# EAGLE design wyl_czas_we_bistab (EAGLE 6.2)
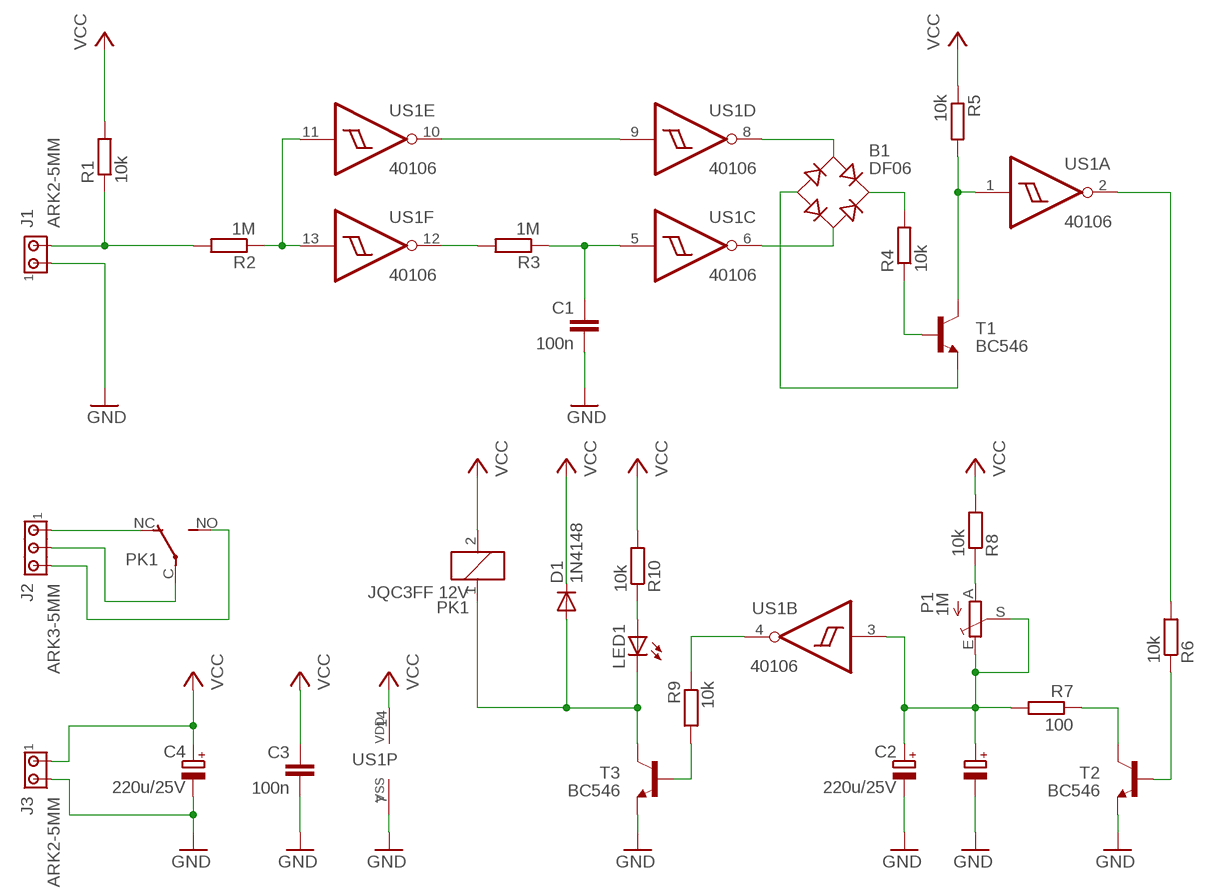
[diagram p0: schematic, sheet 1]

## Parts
B1  DF06  B-DIL  [B-DIL]
C1  100n  C-EU050-025X075  [C050-025X075]
C2  220u/25V  CPOL-EUE2.5-7  [E2,5-7]
C2'  CPOL-EUE5-10.5  [E5-10,5]
C3  100n  C-EU050-025X075  [C050-025X075]
C4  220u/25V  CPOL-EUE2.5-7  [E2,5-7]
D1  1N4148  1N4148DO35-7  [DO35-7]
J1  ARK2-5MM  [2PIN-5MM]
J2  ARK3-5MM  [3PIN-5MM]
J3  ARK2-5MM  [2PIN-5MM]
LED1  LED5MM  [LED5MM]
P1  1M  TRIM_EU-CA6V  [CA6V]
PK1  JQC3FF 12V  PK_POJED-JQC-3FG  [PK_POJED_JQC-3FG]
R1  10k  R-EU_0207/7  [0207/7]
R2  1M  R-EU_0207/7  [0207/7]
R3  1M  R-EU_0207/7  [0207/7]
R4  10k  R-EU_0207/2V  [0207/2V]
R5  10k  R-EU_0207/7  [0207/7]
R6  10k  R-EU_0207/2V  [0207/2V]
R7  100  R-EU_0207/2V  [0207/2V]
R8  10k  R-EU_0207/10  [0207/10]
R9  10k  R-EU_0207/2V  [0207/2V]
R10  10k  R-EU_0207/7  [0207/7]
T1  BC546  BC546B  [TO92-EBC]
T2  BC546  BC546B  [TO92-EBC]
T3  BC546  BC546B  [TO92-EBC]
US1  40106  40106N  [DIL14]

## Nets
GND: C1.2 C2'.- C2.- C3.2 C4.- J1.P$1 J3.P$2 T2.E T3.E US1.7(P:VSS)
J2: J2.P$2 PK1.C(COM)
N$1: B1.AC1 US1.8(D:O)
N$2: B1.+ R4.2
N$3: B1.AC2 US1.6(C:O)
N$4: R9.1 US1.4(B:O)
N$5: R4.1 T1.B
N$6: J1.P$2 R1.1 R2.2
N$7: R9.2 T3.B
N$8: LED1.A R10.1
N$9: J2.P$1 PK1.NC
N$10: R2.1 US1.11(E:I) US1.13(F:I)
N$11: J2.P$3 PK1.NO
N$12: R3.2 US1.12(F:O)
N$13: C1.1 R3.1 US1.5(C:I)
N$14: B1.- T1.E
N$15: R5.2 T1.C US1.1(A:I)
N$16: US1.9(D:I) US1.10(E:O)
N$17: R6.2 US1.2(A:O)
N$18: R6.1 T2.B
N$19: R7.1 T2.C
N$20: C2'.+ C2.+ P1.E P1.S R7.2 US1.3(B:I)
N$21: P1.A R8.1
N$22: D1.A LED1.K(C) PK1.1 T3.C
VCC: C3.1 C4.+ D1.C J3.P$1 PK1.2 R1.2 R5.1 R8.2 R10.2 US1.14(P:VDD)

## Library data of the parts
B1 = rectifier:B-DIL: RECTIFIER
C1 C3 = rcl:C-EU: CAPACITOR, European symbol
C2 C2' C4 = rcl:CPOL-EU: POLARIZED CAPACITOR, European symbol
D1 = diode:1N4148: DIODE
J1 J3 = zlacza_futrzak:ARK2: ARK 2
J2 = zlacza_futrzak:ARK3: ARK 3 Raster 5mm i 3,5mm
LED1 = led:LED: LED
P1 = pot:TRIM_EU-: POTENTIOMETER
PK1 = inne_futrzak:PK_POJED
R1-R10 = rcl:R-EU_: RESISTOR, European symbol
T1-T3 = transistor-npn:BC546*: NPN Transistor
US1 = 40xx:40106: Hex SCHMITT TRIGGER

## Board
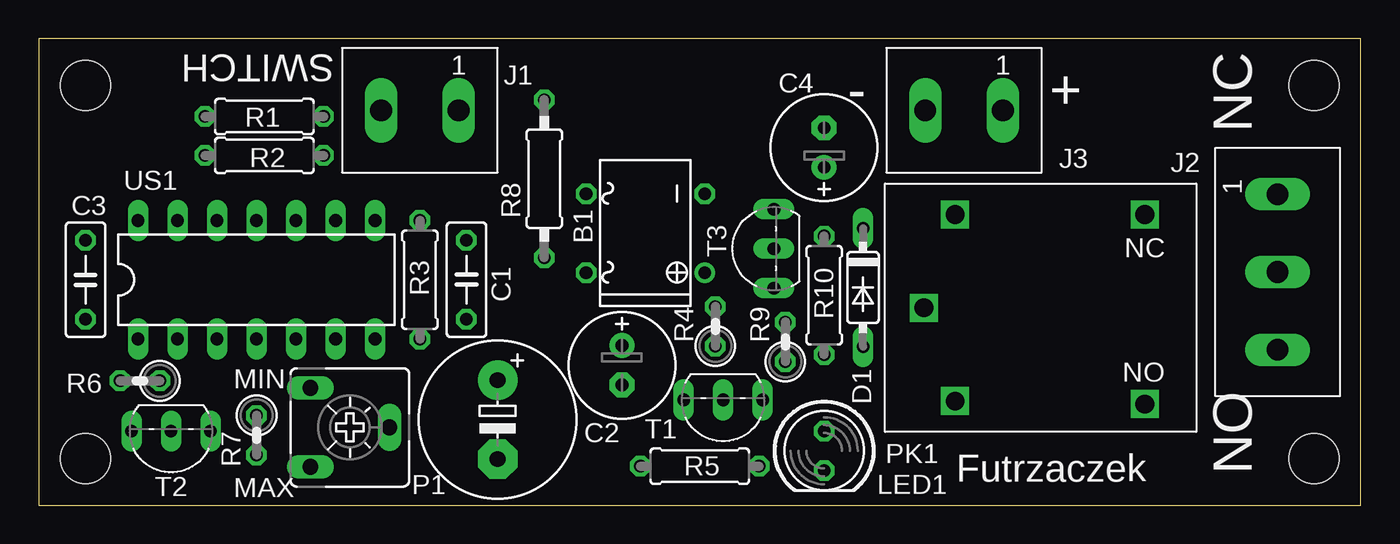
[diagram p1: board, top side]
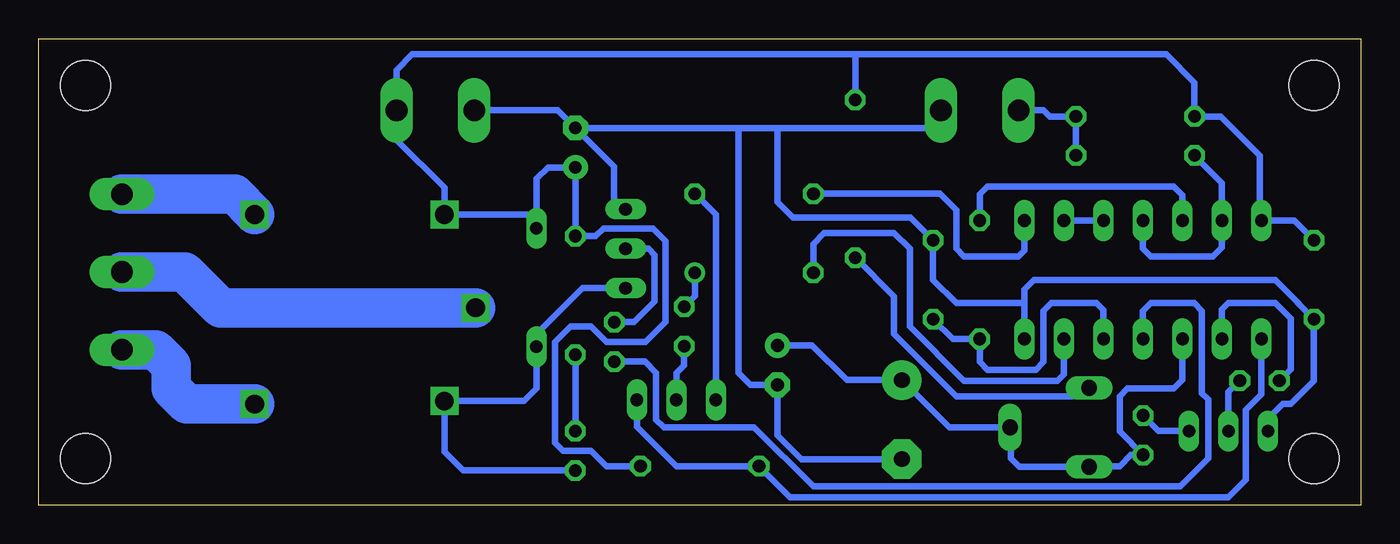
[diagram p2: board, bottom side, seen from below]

Size 85 x 30 mm. Coordinates in mm from the lower left corner, seen from the top.
Outline: 0,0 85,0 85,30 0,30 0,0
Copper layers (1*16): Top 0.035mm / dielectric 1.5mm / Bottom 0.035mm
Design rules: minimum track width 10mil, minimum drill 23mil, track to track 8mil, track to pad 8mil, pad to pad 8mil, via to via 8mil, smd to smd 8mil, copper to edge 10mil, drill to drill 8mil, minimum pad ring 10mil, minimum via ring 8mil, stop-mask expansion 4mil, vias tented up to drill 0mil, thermal gap 10mil
Holes 3.2 mm at 3,3 3,27 82,3 82,27

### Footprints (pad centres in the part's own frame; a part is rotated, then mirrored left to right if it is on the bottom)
B-DIL = drill 0.813: + -2.54,-3.81 | drill 0.813 octagon: - 2.54,-3.81; AC1 2.54,3.81; AC2 -2.54,3.81
C050-025X075 = drill 0.813 octagon: 1 -2.54,0; 2 2.54,0
E2,5-7 = drill 0.813 pad 1.6: + -1.27,0 | drill 0.813 pad 1.6 octagon: - 1.27,0
E5-10,5 = drill 1.016 pad 2.54: + -2.54,0 | drill 1.016 pad 2.54 octagon: - 2.54,0
DO35-7 = drill 0.813 long: A 3.81,0; C -3.81,0
2PIN-5MM = drill 1.4 long: P$1 -2.5,0; P$2 2.5,0
3PIN-5MM = drill 1.4 long: P$1 -5,0; P$2 0,0; P$3 5,0
LED5MM = drill 0.813 octagon: A -1.27,0; K 1.27,0
CA6V = drill 1.016 long: A -2.54,-2.54; E 2.54,-2.54; S 0,2.54
PK_POJED_JQC-3FG = drill 1.2 square: 1 5.5,6; 2 5.5,-6; C 7.5,0; NC -6.7,-6; NO -6.7,6.2
0207/7 = drill 0.813 octagon: 1 -3.81,0; 2 3.81,0
0207/2V = drill 0.813 octagon: 1 -1.27,0; 2 1.27,0
0207/10 = drill 0.813 octagon: 1 -5.08,0; 2 5.08,0
TO92-EBC = drill 0.813 long: B 0,-1.27; C -2.54,-1.27; E 2.54,-1.27
DIL14 = drill 0.813 long: 1 -7.62,-3.81; 2 -5.08,-3.81; 3 -2.54,-3.81; 4 0,-3.81; 5 2.54,-3.81; 6 5.08,-3.81; 7 7.62,-3.81; 8 7.62,3.81; 9 5.08,3.81; 10 2.54,3.81; 11 0,3.81; 12 -2.54,3.81; 13 -5.08,3.81; 14 -7.62,3.81

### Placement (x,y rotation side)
B1  39,17.5 90 top
C1  27.5,14.5 90 top
C2  37.5,9 270 top
C2'  29.5,5.5 270 top
C3  3,14.5 270 top
C4  50.5,23 90 top
D1  53,14 270 top
J1  24.5,25.4 180 top
J2  79.66,15 270 top
J3  59.5,25.4 180 top
LED1  50.5,3.5 270 top
P1  20,5 270 top
PK1  64.42,12.7 180 top
R1  14.5,25 180 top
R2  14.5,22.5 0 top
R3  24.5,14.5 90 top
R4  43.5,11.5 90 top
R5  42.5,2.5 180 top
R6  6.5,8 180 top
R7  14,4.5 270 top
R8  32.5,21 90 top
R9  48,10.5 90 top
R10  50.5,13.5 90 top
T1  44,5.5 180 top
T2  8.5,3.5 180 top
T3  46,16.5 90 top
US1  14,14.5 0 top

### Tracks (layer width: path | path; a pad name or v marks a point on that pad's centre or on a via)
GND
  Bottom 0.406: J1.P$1 27,24.5 27.5,24.5 27.77,24.27 37.5,24.27 | T3.E 47.54,19.04 48,19.5 48,21.77 C4.- | US1.7 21.62,13 | 21.62,13 26,13 27.5,14.5 C1.2 28.96,18.5 36.5,18.5 37.5,19.5 37.5,22.64 37.5,24.27 | 21.62,13 21.62,13.88 21,14.5 5.5,14.5 4,13 4.04,13 C3.2 3,8 4.5,6.5 5,6.5 5.96,5.54 T2.E | C2'.- 35.96,2.96 37.5,4.5 C2.- 39.23,7.73 40,8.5 40,23.14 40,24.27 | C4.- 40,24.27 | 40,24.27 37.5,24.27 | J3.P$2 51.63,25.4 C4.-
J2
  Bottom 2.54: PK1.C 73.31,12.7 75.61,15 J2.P$2
N$1
  Bottom 0.406: US1.8 21.62,16.38 22,16 25.5,16 26,16.5 26,19 27.04,20.04 B1.AC1
N$2
  Bottom 0.406: B1.+ 42.81,13.46 R4.2
N$3
  Bottom 0.406: US1.6 19.08,8.42 19.5,8 25.5,8 29,11.5 29,16.5 30,17.5 34.5,17.5 35.19,16.81 B1.AC2
N$4
  Bottom 0.406: US1.4 14,12.5 13.5,13 10.7,13 10.2,12.5 10.2,7.2 9.8,6.8 9.8,3 11.6,1.2 35.2,1.2 39,5 44.8,5 45.3,5.5 45.3,8.5 46.03,9.23 R9.1
N$5
  Bottom 0.406: T1.B 44,8.5 43.5,9 R4.1
N$6
  Bottom 0.406: J1.P$2 20.4,25.4 20,25 R1.1 R2.2
N$7
  Bottom 0.406: T3.B 45.8,16.5 45.4,16.1 45.4,13.1 46.73,11.77 R9.2
N$8
  Bottom 0.406: LED1.A R10.1
N$9
  Bottom 2.54: J2.P$1 72.42,20 PK1.NC
N$10
  Bottom 0.406: R2.1 8.92,20.73 US1.13 8.92,16.58 9.5,16 13.5,16 14,16.5 US1.11
N$11
  Bottom 2.54: PK1.NO 75.5,6.5 76.5,7.5 76.5,9 77.5,10 J2.P$3
N$12
  Bottom 0.406: R3.2 24.5,20 24,20.5 12,20.5 11.46,19.96 US1.12
N$13
  Bottom 0.406: C1.1 26.23,10.69 R3.1 24.5,9.2 24,8.7 20.9,8.7 20.4,9.2 20.4,12.5 19.9,13 17,13 16.54,12.54 US1.5
N$14
  Bottom 0.406: T1.E 41.46,18.69 B1.-
N$15
  Bottom 0.406: T1.C 46.54,5.04 44,2.5 R5.2 36.69,0.5 8.5,0.5 7.38,1.62 7.38,6.12 6.38,7.12 US1.1
N$16
  Bottom 0.406: US1.10 US1.9
N$17
  Bottom 0.406: US1.2 8.92,12.58 8.5,13 5.5,13 4.5,12 4.5,8.73 R6.2
N$18
  Bottom 0.406: T2.B 8.5,7.27 R6.1
N$19
  Bottom 0.406: T2.C 13,4.77 R7.1
N$20
  Bottom 0.406: C2.+ 35.27,10.27 33.04,8.04 C2'.+ 26.46,5 P1.S 22.5,4.96 22.5,3 21.96,2.46 P1.E 17.42,2.5 15.5,2.5 14.77,3.23 R7.2 15.5,4.73 15.5,7 15,7.5 12,7.5 11.46,8.04 US1.3
N$21
  Bottom 0.406: P1.A 17.96,7.54 18.5,7 26,7 30,11 30,13.42 R8.1
N$22
  Bottom 0.406: LED1.K 57.73,2.23 58.92,3.42 PK1.1 53.8,6.7 53,7.5 D1.A 53,11 50.04,13.96 T3.C
VCC
  Bottom 0.406: 32.5,29 61,29 62,28 J3.P$1 62,23.5 58.92,20.42 PK1.2 53.2,18.7 53,18 D1.C 53,21 52.27,21.73 C4.+ R10.2 49.19,17.31 48.7,17.8 45.5,17.8 44.7,17 44.7,11.8 46,10.5 48.5,10.5 49.5,11.5 50.8,11.5 51.8,10.5 51.8,4 51.3,3.5 49.5,3.5 48.5,2.5 R5.1 | 32.5,29 12.5,29 10.69,27.19 R1.2 9,25 6.5,22.5 6.5,18.43 US1.14 4.27,18.31 C3.1 | R8.2 32.5,29

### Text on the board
tPlace: SWITCH | - | + | NC | MIN | Futrzaczek | NO | MAX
